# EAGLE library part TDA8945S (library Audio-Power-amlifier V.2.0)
The TDA8945S is a single-channel audio power amplifier with an output power of 15 W at an 8 W load and an 18 V supply. The circuit contains a Bridge Tied Load (BTL) amplifier with an all-NPN output stage and standby/mute logic. The TDA8945S comes in a 9-lead single in-line (SIL) power package. The TDA8945S is printed-circuit board (PCB) compatible with all other types in the TDA894x family. One PCB footprint accommodates both the mono and the stereo products.
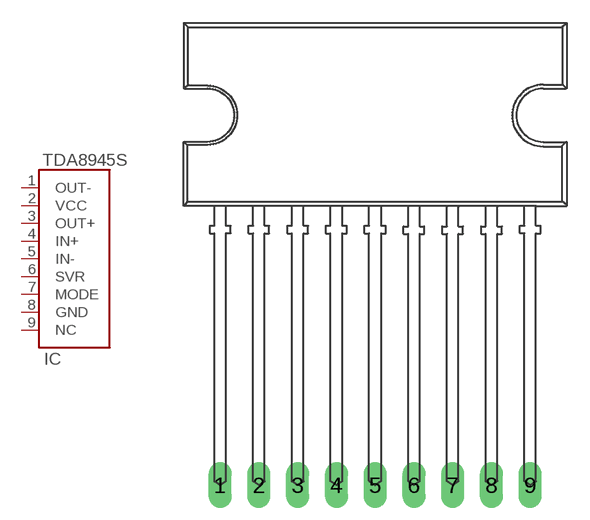
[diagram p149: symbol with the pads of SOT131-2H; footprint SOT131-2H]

Designator prefix IC

## TDA8945S  [SOT131-2H]
1  OUT-  out
2  VCC  pwr
3  OUT+  out
4  IN+  in
5  IN-  in
6  SVR
7  MODE
8  GND  pwr
9  NC  nc

## Footprint SOT131-2H (pad centres in mm)
drill 1 long: 1 -10.16,0; 2 -7.62,0; 3 -5.08,0; 4 -2.54,0; 5 0,0; 6 2.54,0; 7 5.08,0; 8 7.62,0; 9 10.16,0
